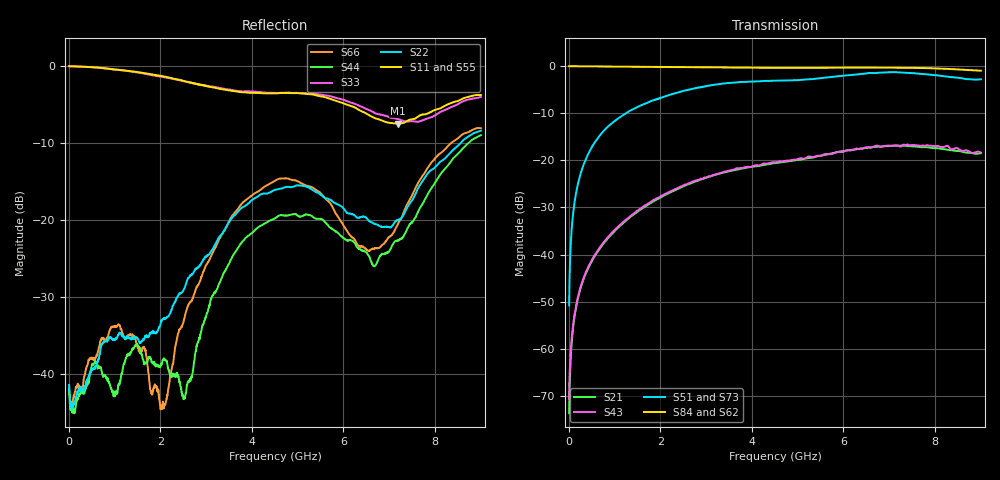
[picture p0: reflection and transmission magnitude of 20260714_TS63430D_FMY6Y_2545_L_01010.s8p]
# GHz S DB R 50
! CMT, SN0916, 25263762, 26.7.0
! Date: 15.07.2026 14:56:54
! Data: Format
! Freq S1.1:dB/Ang S1.2:dB/Ang S1.3:dB/Ang S1.4:dB/Ang S1.5:dB/Ang S1.6:dB/Ang S1.7:dB/Ang S1.8:dB/Ang
!  S2.1:dB/Ang S2.2:dB/Ang S2.3:dB/Ang S2.4:dB/Ang S2.5:dB/Ang S2.6:dB/Ang S2.7:dB/Ang S2.8:dB/Ang
!  S3.1:dB/Ang S3.2:dB/Ang S3.3:dB/Ang S3.4:dB/Ang S3.5:dB/Ang S3.6:dB/Ang S3.7:dB/Ang S3.8:dB/Ang
!  S4.1:dB/Ang S4.2:dB/Ang S4.3:dB/Ang S4.4:dB/Ang S4.5:dB/Ang S4.6:dB/Ang S4.7:dB/Ang S4.8:dB/Ang
!  S5.1:dB/Ang S5.2:dB/Ang S5.3:dB/Ang S5.4:dB/Ang S5.5:dB/Ang S5.6:dB/Ang S5.7:dB/Ang S5.8:dB/Ang
!  S6.1:dB/Ang S6.2:dB/Ang S6.3:dB/Ang S6.4:dB/Ang S6.5:dB/Ang S6.6:dB/Ang S6.7:dB/Ang S6.8:dB/Ang
!  S7.1:dB/Ang S7.2:dB/Ang S7.3:dB/Ang S7.4:dB/Ang S7.5:dB/Ang S7.6:dB/Ang S7.7:dB/Ang S7.8:dB/Ang
!  S8.1:dB/Ang S8.2:dB/Ang S8.3:dB/Ang S8.4:dB/Ang S8.5:dB/Ang S8.6:dB/Ang S8.7:dB/Ang S8.8:dB/Ang
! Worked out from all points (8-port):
!   2001 points, 10 MHz to 9 GHz, reference 50 ohm
!   strongest paths, dB at 10 MHz, 2.257 GHz, 4.505 GHz, 6.753 GHz, 9 GHz:
!     S84: -0.1, -0.3, -0.4, -0.4, -1.0
!     S62: -0.1, -0.3, -0.5, -0.5, -1.2
!     S51: -50.8, -6.0, -3.2, -1.5, -2.8
!     S73: -51.3, -6.1, -3.4, -1.7, -2.8
!     S43: -70.7, -26.5, -20.5, -17.0, -18.4
!     S21: -73.7, -26.6, -20.6, -17.2, -18.5
!   lowest |S11| = -7.5 dB at 7.18 GHz (marker M1), VSWR 2.46, Z = 21.2 - j9.55 ohm
!   |S11| at or under -10 dB: nowhere
